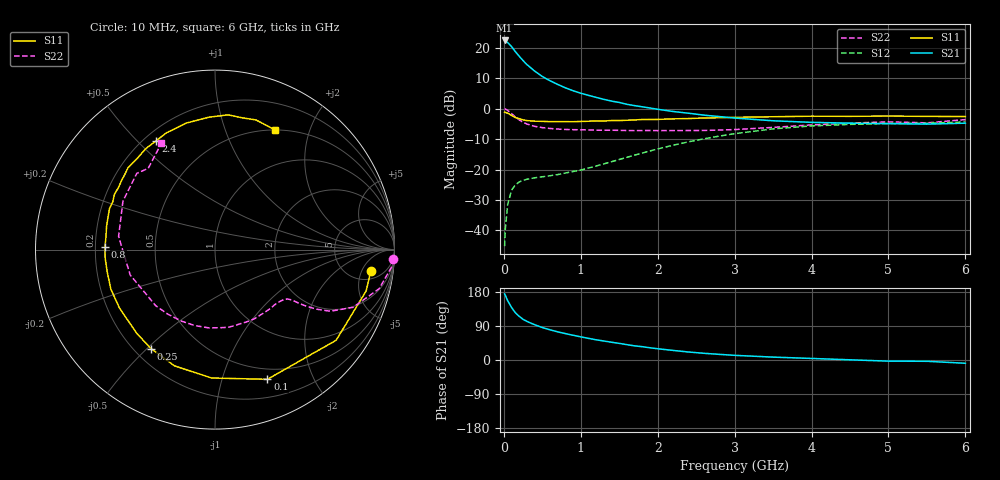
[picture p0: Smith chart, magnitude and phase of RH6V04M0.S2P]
! SIEMENS Small Signal Semiconductors
! BFR106
! Si NPN RF Bipolar Junction Transistor in SOT23
! VCE = 6 V  IC = 4 mA
! Common Emitter S-Parameters:  August  1996
# GHz  S  MA  R  50
!  f  S11  S21  S12  S22
! GHz  MAG  ANG  MAG  ANG  MAG  ANG  MAG  ANG
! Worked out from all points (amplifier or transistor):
!   36 points, 10 MHz to 6 GHz, reference 50 ohm
!   highest |S21| = 22.5 dB at 10 MHz (marker M1)
!   |S21| within 3 dB of that: start of sweep to 129.8 MHz
!   unconditionally stable (mu >= 1): 669.2 MHz to 1.807 GHz; 4.675 GHz to end of sweep
!   at 250 MHz: K = 0.45, MSG = 19.7 dB, |S12| = -23.6 dB
!   at 1.4 GHz: K = 1.14, MAG = 7.7 dB, |S12| = -17.4 dB
!   at 6 GHz: K = 1.02, MAG = -1.0 dB, |S12| = -4.3 dB
!   S11 on the Smith chart (normalised r, x): 10 MHz: 7, -8; 100 MHz: 0.38, -1.41; 250 MHz: 0.27, -0.51; 800 MHz: 0.24, +0.01; 2.4 GHz: 0.25, +0.57; 6 GHz: 0.50, +1.50
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0.01  0.8766 -7.8  13.26 174.4  0.0055 86.6  0.9946 -2.9
0.02  0.8729 -15.3  13.12 170.4  0.0108 82.3  0.988 -5.7
0.05  0.8431 -36.8  12.24 156.5  0.0267 71.0  0.9402 -13.4
0.1  0.7794 -68.0  10.54 138.8  0.0457 57.3  0.8335 -22.7
0.15  0.7157 -91.5  8.685 124.5  0.0562 47.6  0.7287 -28.1
0.2  0.6859 -109.2  7.297 115.2  0.0625 42.3  0.656 -30.4
0.25  0.6569 -122.9  6.187 107.3  0.0664 38.7  0.598 -31.8
0.3  0.6382 -133.2  5.33 101.8  0.0693 37.5  0.561 -32.5
0.4  0.624 -148.6  4.164 93.1  0.0731 36.8  0.5141 -33.2
0.5  0.6206 -159.3  3.391 85.7  0.0761 38.2  0.4891 -34.2
0.6  0.6132 -168.4  2.888 79.7  0.0792 40.7  0.4738 -36.0
0.8  0.6133 178.5  2.208 69.7  0.0877 47.1  0.4564 -40.6
0.9  0.6116 173.4  1.976 65.3  0.0929 50.5  0.4527 -42.9
1.1  0.623 163.0  1.661 57.1  0.1058 56.6  0.4476 -49.4
1.6  0.6468 143.7  1.182 40.5  0.1588 65.6  0.4387 -67.7
2.2  0.6818 124.5  0.901 25.3  0.2513 64.3  0.4376 -94.2
2.4  0.6893 118.4  0.844 21.1  0.2857 61.8  0.4381 -104.9
3.5  0.7383 92.7  0.634 7.6  0.4665 41.3  0.4933 -163.4
4.5  0.75 78.0  0.579 0.5  0.5528 20.3  0.5797 152.2
5  0.7575 72.5  0.569 -3.0  0.5712 11.7  0.6085 135.7
5.5  0.7488 66.9  0.558 -3.4  0.5768 7.3  0.586 129.4
6  0.7442 63.4  0.579 -8.6  0.6064 -0.9  0.6631 116.8
